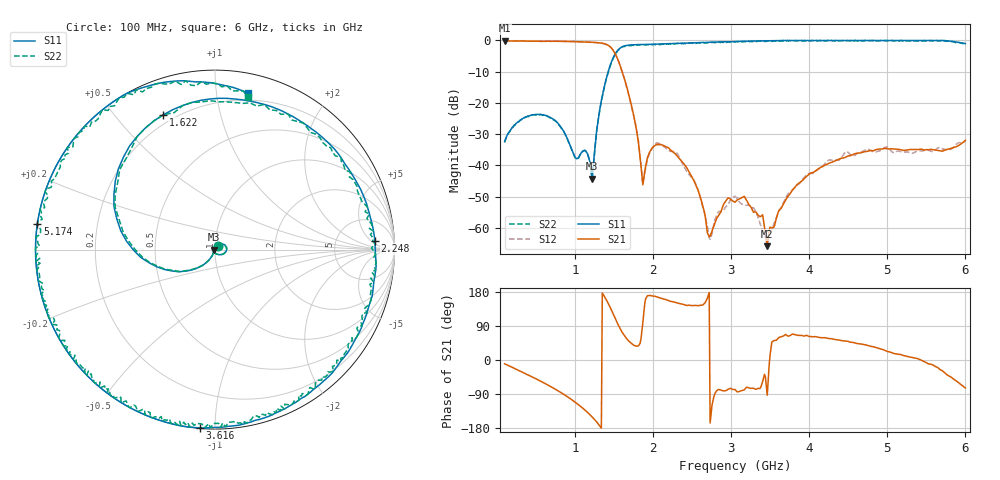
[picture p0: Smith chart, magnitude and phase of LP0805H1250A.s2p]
!	AVX	THIN	FILM	OPERATION
!	LP0805	High	Performance	Low	Pass	Filter	P/N	LP0805H1250ASTR
!	29	June	2017
#	MHz	S	dB	R	50
!	Frq	S11(dB)	S11(deg)	S21(dB)	S21(deg)	S12(dB)	S12(deg)	S22(dB)	S22(deg)
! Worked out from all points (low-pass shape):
!   501 points, 100 MHz to 6 GHz, reference 50 ohm
!   highest |S21| = -0.11 dB at 100 MHz (marker M1); lowest = -65.9 dB at 3.463 GHz (marker M2)
!   |S21| within 3 dB of the highest: start of sweep to 1.488 GHz
!   lowest |S11| = -44.3 dB at 1.221 GHz (marker M3), VSWR 1.01, Z = 49.4 + j0.00464 ohm
!   |S11| at or under -10 dB: start of sweep to 1.427 GHz
!   |S22| runs from -44.4 to 0.0 dB; largest |S21 - S12| = 0.024
!   S11 on the Smith chart (normalised r, x): 100 MHz: 1.03, +0.04; 1.622 GHz: 0.16, +0.68; 2.248 GHz: 14, +7; 3.616 GHz: 0.00, -0.92; 5.174 GHz: 0.00, +0.07; 6 GHz: 0.14, +1.22
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100  -32.40 50.6  -0.11 -10.0  -0.10 -10.0  -32.60 50.4
572  -23.72 0.1  -0.29 -56.9  -0.29 -57.0  -23.72 -0.0
1091.2  -35.70 156.4  -0.45 -125.5  -0.45 -125.7  -35.70 156.2
1221  -44.27 179.6  -0.59 -150.3  -0.62 -150.5  -44.37 179.6
1327.2  -20.91 -124.4  -0.79 -176.4  -0.83 -176.7  -21.01 -124.5
1468.8  -6.84 -179.8  -2.48 131.3  -2.48 129.5  -7.04 -180.0
1622.2  -1.89 110.9  -11.34 68.1  -11.42 70.5  -1.89 110.8
1787.4  -1.34 66.3  -28.54 36.7  -28.16 38.0  -1.44 66.1
1870  -1.29 51.0  -46.21 98.5  -45.95 101.3  -1.49 50.8
2070.6  -1.13 22.6  -33.37 165.0  -32.91 163.3  -1.33 22.4
2247.6  -1.00 3.2  -35.53 154.1  -35.58 156.1  -1.10 3.2
2542.6  -0.74 -23.3  -45.96 144.1  -45.62 140.0  -0.94 -23.3
2731.4  -0.57 -38.0  -62.72 -166.4  -63.63 -147.2  -0.67 -38.2
3050  -0.37 -60.0  -51.79 -77.7  -49.84 -76.0  -0.57 -60.2
3380.4  -0.13 -80.9  -56.34 -71.9  -59.37 -71.2  -0.13 -80.9
3463  -0.11 -85.8  -65.86 -92.9  -64.73 -31.5  -0.21 -86.0
3616.4  -0.03 -94.8  -54.30 59.8  -54.34 62.4  -0.23 -94.8
4041.2  0.00 -118.8  -42.29 61.5  -42.55 63.1  0.00 -118.8
5020.6  0.00 -176.9  -34.73 21.8  -34.55 19.3  -0.20 -177.1
5174  0.00 171.8  -35.02 14.2  -35.61 10.3  0.00 171.8
5598.8  0.00 133.0  -35.01 -15.0  -35.38 -11.2  -0.20 132.8
6000  -1.00 78.0  -31.99 -73.7  -32.12 -68.0  -1.20 77.9
